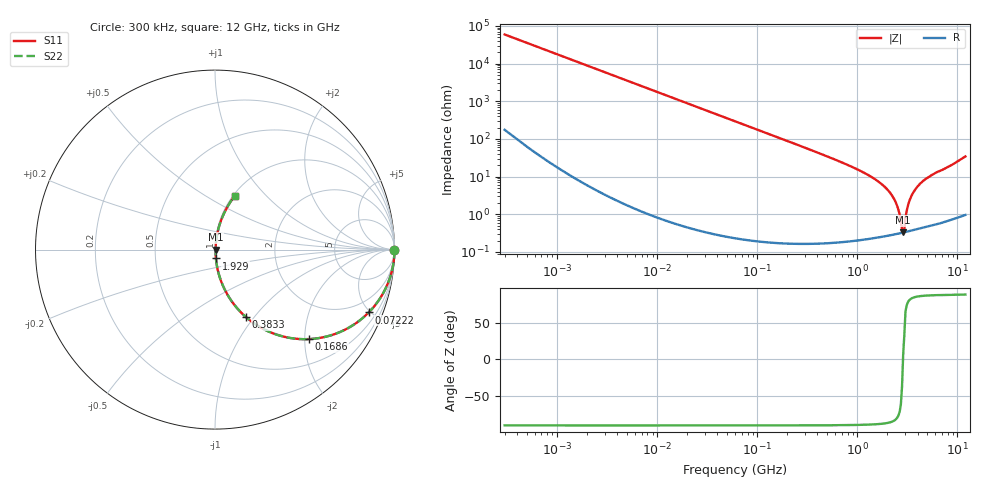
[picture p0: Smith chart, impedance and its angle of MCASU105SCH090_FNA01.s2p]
! MCASU105SCH090_FNA01  S-PARAMETER MODEL  ( Standard Model )
! Model Generated by TAIYO YUDEN Corporation (http://www.ty-top.com)
! Version 1.0
! TAIYO YUDEN Control No. 230609
! Copyright(c) 2023 TAIYO YUDEN CO.,LTD. All Rights Reserved.
! Product Description (link to TY-COMPAS)
! https://ds.yuden.co.jp/TYCOMPAS/or/detail?pn=MCASU105SCH090CFNA01&u=M
! Products Name : Multilayer Ceramic Capacitors
! Characteristics :
!  Capacitance : 9 [pF] , Rated Voltage : 50 [V] , TCC : CH / C0H
!  Case Size : 1.0 x 0.5 / 0.039 x 0.02 [mm/inch] , Thickness : 0.5 / 0.02 [mm/inch]
!  (Conditions: Temperature = 25 [degC] , DC Bias Voltage = 0 [V])
! External Node Assignments :
!  1  o---| |---o  2
! GND o---------o GND
! Frequency Range : 0.3MHz  -  12000MHz  [ 401 STEP ]
# MHZ S RI R 50
! Freq[MHz].  S11 Real  S11 Imag  S21 Real  S21 Imag  S12 Real  S12 Imag  S22 Real  S22 Imag
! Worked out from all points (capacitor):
!   401 points, 300 kHz to 12 GHz, reference 50 ohm
!   read as one part in series: C = 9 pF near 316.3 kHz
!   lowest |Z| = 329 mohm at 2.87 GHz (marker M1)
!   series resonance near 2.86 GHz, so ESL is about 340 pH
!   S11 on the Smith chart (normalised r, x): 300 kHz: open; 72.22 MHz: 1.00, -4.89; 168.6 MHz: 1.00, -2.09; 383.3 MHz: 1.00, -0.91; 1.929 GHz: 1.01, -0.10; 12 GHz: 1.02, +0.68
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0.3  1 -0.0017  7.89e-06 0.0017  7.89e-06 0.0017  1 -0.0017
1.769972  0.9999 -0.01  0.000107 0.01  0.000107 0.01  0.9999 -0.01
10.44266  0.9965 -0.0588  0.0035 0.0588  0.0035 0.0588  0.9965 -0.0588
26.39317  0.9781 -0.146  0.0219 0.146  0.0219 0.146  0.9781 -0.146
60  0.8965 -0.3042  0.1035 0.3042  0.1035 0.3042  0.8965 -0.3042
72.22496  0.8567 -0.35  0.1433 0.35  0.1433 0.35  0.8567 -0.35
168.5979  0.5221 -0.4987  0.4779 0.4987  0.4779 0.4987  0.5221 -0.4987
353.9943  0.1956 -0.395  0.8044 0.395  0.8044 0.395  0.1956 -0.395
383.2761  0.1712 -0.3749  0.8288 0.3749  0.8288 0.3749  0.1712 -0.3749
1076.992  0.0214 -0.1375  0.9786 0.1375  0.9786 0.1375  0.0214 -0.1375
1928.972  0.00507 -0.0493  0.9949 0.0493  0.9949 0.0493  0.00507 -0.0493
2088.533  0.00425 -0.0389  0.9957 0.0389  0.9957 0.0389  0.00425 -0.0389
2448.343  0.00333 -0.0188  0.9967 0.0188  0.9967 0.0188  0.00333 -0.0188
2795.104  0.00321 -0.00241  0.9968 0.00241  0.9968 0.00241  0.00321 -0.00241
2870.14  0.00326 0.000384  0.9967 -0.000384  0.9967 -0.000384  0.00326 0.000384
2947.191  0.00332 0.0022  0.9967 -0.0022  0.9967 -0.0022  0.00332 0.0022
3190.978  0.00374 0.0159  0.9963 -0.0159  0.9963 -0.0159  0.00374 0.0159
3364.605  0.00423 0.0248  0.9958 -0.0248  0.9958 -0.0248  0.00423 0.0248
3642.919  0.00528 0.0383  0.9947 -0.0383  0.9947 -0.0383  0.00528 0.0383
4158.869  0.00786 0.0606  0.9921 -0.0606  0.9921 -0.0606  0.00786 0.0606
5715.274  0.018 0.1124  0.982 -0.1124  0.982 -0.1124  0.018 0.1124
12000  0.1113 0.3008  0.8887 -0.3008  0.8887 -0.3008  0.1113 0.3008
